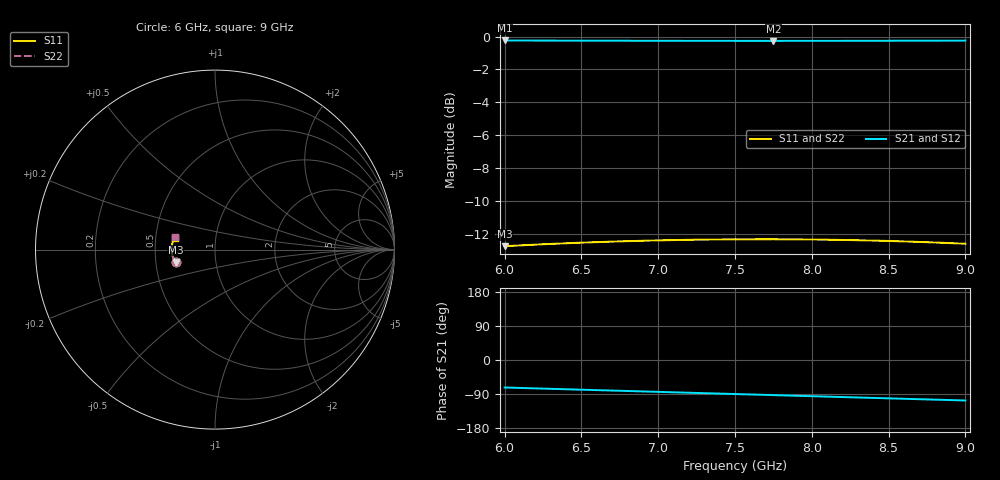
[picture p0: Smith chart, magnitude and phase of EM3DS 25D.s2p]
!AWR Design Environment (2469) Mon Oct 04 18:05:22 2004
!freq-unit  param-type  data-format  keyword  impedance-ohms
# GHz  S  MA  R  50
!Freq  MagS11  AngS11  MagS21  AngS21  MagS12  AngS12  MagS22  AngS22
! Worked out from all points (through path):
!   13 points, 6 GHz to 9 GHz, reference 50 ohm
!   highest |S21| = -0.24 dB at 6 GHz (marker M1); lowest = -0.3 dB at 7.75 GHz (marker M2)
!   group delay of S21, straight-line fit = 31.7 ps
!   lowest |S11| = -12.7 dB at 6 GHz (marker M3), VSWR 1.60, Z = 31.7 - j4.62 ohm
!   |S11| at or under -10 dB: start of sweep to end of sweep
!   |S22| runs from -12.7 to -12.3 dB; largest |S21 - S12| = 0
6  0.2304 -162.6  0.9731 -72.6  0.9731 -72.6  0.2304 -162.6
6.25  0.2336 -165.5  0.9724 -75.5  0.9724 -75.5  0.2336 -165.5
6.5  0.2362 -168.3  0.9717 -78.3  0.9717 -78.3  0.2362 -168.4
6.75  0.2383 -171.2  0.9712 -81.2  0.9712 -81.2  0.2383 -171.2
7  0.24 -174.0  0.9708 -84.1  0.9708 -84.1  0.24 -174.1
7.25  0.2411 -176.9  0.9705 -86.9  0.9705 -86.9  0.2411 -177.0
7.5  0.2418 -179.7  0.9703 -89.8  0.9703 -89.8  0.2418 -179.9
7.75  0.2419 177.5  0.9703 -92.7  0.9703 -92.7  0.2419 177.2
8  0.2415 174.7  0.9704 -95.5  0.9704 -95.5  0.2415 174.3
8.25  0.2405 171.9  0.9707 -98.3  0.9707 -98.3  0.2405 171.4
8.5  0.239 169.2  0.971 -101.2  0.971 -101.2  0.239 168.5
8.75  0.2369 166.4  0.9715 -104.0  0.9715 -104.0  0.2369 165.5
9  0.2344 163.7  0.9721 -106.9  0.9721 -106.9  0.2344 162.6
